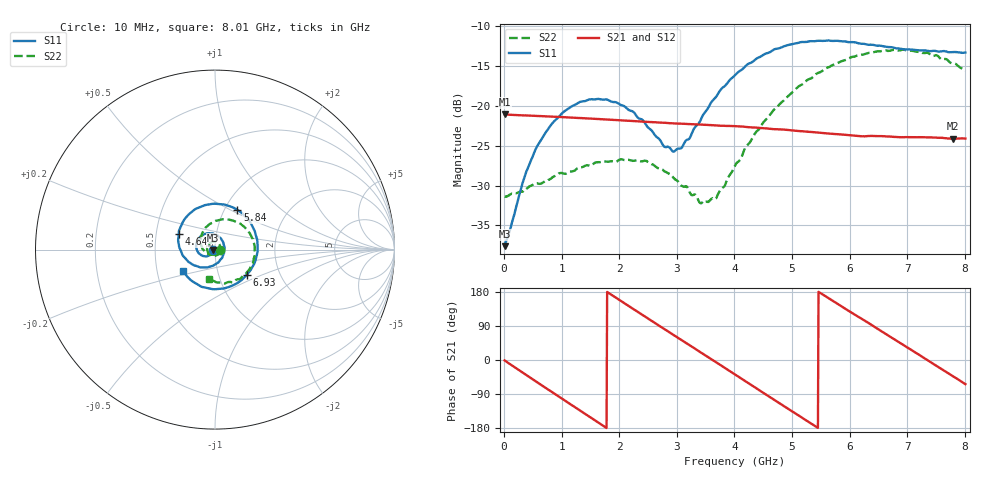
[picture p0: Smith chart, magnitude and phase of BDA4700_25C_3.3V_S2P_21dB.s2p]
!Agilent Technologies,E5071B,MY42404982,A.09.10
!Date: Mon Oct 20 18:11:52 2025
!Data & Calibration Information:
!Freq	S11:SOLT2(ON)	S21:SOLT2(ON)	S12:SOLT2(ON)	S22:SOLT2(ON)
# Hz S RI R 50
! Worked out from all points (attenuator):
!   801 points, 10 MHz to 8.01 GHz, reference 50 ohm
!   highest |S21| = -21.08 dB at 20 MHz (marker M1); lowest = -24.1 dB at 7.8 GHz (marker M2)
!   lowest |S11| = -37.6 dB at 10 MHz (marker M3), VSWR 1.03, Z = 48.7 - j0.141 ohm
!   |S11| at or under -10 dB: start of sweep to end of sweep
!   |S22| runs from -32.2 to -13.0 dB; largest |S21 - S12| = 0.00096
!   S11 on the Smith chart (normalised r, x): 10 MHz: 0.97, -0.00; 4.64 GHz: 0.66, +0.12; 5.84 GHz: 1.15, +0.54; 6.93 GHz: 1.37, -0.40; 8.01 GHz: 0.68, -0.17
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1e7  -0.0131 -0.00145  0.0883 -0.00193  0.0883 -0.00194  0.027 -0.000793
2e7  -0.0135 -0.00226  0.0883 -0.0034  0.0882 -0.00366  0.0269 -0.00108
3.5e8  -0.0237 -0.0261  0.0704 -0.0511  0.0704 -0.0511  0.0228 -0.0184
5.8e8  -0.0423 -0.0369  0.0442 -0.0741  0.0441 -0.0741  0.0143 -0.0292
1e9  -0.0857 -0.0243  -0.0169 -0.0832  -0.0168 -0.0832  -0.0149 -0.0349
1.35e9  -0.1054 0.015  -0.0607 -0.0575  -0.0607 -0.0576  -0.037 -0.018
1.97e9  -0.0568 0.0873  -0.0771 0.0255  -0.0772 0.0255  -0.0345 0.0289
2.68e9  0.0446 0.0438  -0.00245 0.0785  -0.00262 0.0785  0.0143 0.038
2.93e9  0.0517 -0.00095  0.0298 0.0717  0.0298 0.0715  0.0261 0.0244
3.06e9  0.0474 -0.0257  0.0449 0.0629  0.0442 0.0632  0.0287 0.0143
3.43e9  -0.002 -0.084  0.0722 0.0242  0.0722 0.0243  0.0199 -0.0143
3.69e9  -0.0586 -0.0987  0.0747 -0.0089  0.0748 -0.00914  0.000688 -0.0266
4.01e9  -0.1354 -0.0763  0.0585 -0.0461  0.0585 -0.0459  -0.0324 -0.0267
4.64e9  -0.202 0.0859  -0.0127 -0.0704  -0.0125 -0.0706  -0.0797 0.0411
5.35e9  -0.0484 0.2491  -0.0673 -0.0125  -0.0672 -0.0129  -0.0158 0.1491
5.84e9  0.1243 0.2217  -0.0532 0.0393  -0.0529 0.0394  0.0949 0.1633
6.26e9  0.2219 0.1016  -0.0159 0.0623  -0.0149 0.0625  0.1839 0.1028
6.68e9  0.2262 -0.0569  0.0284 0.0575  0.0286 0.0574  0.221 -0.00237
6.93e9  0.1781 -0.1391  0.0485 0.0409  0.0487 0.0407  0.2128 -0.0723
7.36e9  0.0353 -0.2178  0.0633 -0.00131  0.0634 -0.00133  0.1383 -0.1636
7.8e9  -0.1255 -0.1771  0.0452 -0.0427  0.0451 -0.0428  0.0167 -0.1836
8.01e9  -0.1783 -0.1213  0.0276 -0.0559  0.0278 -0.0559  -0.0331 -0.1621
